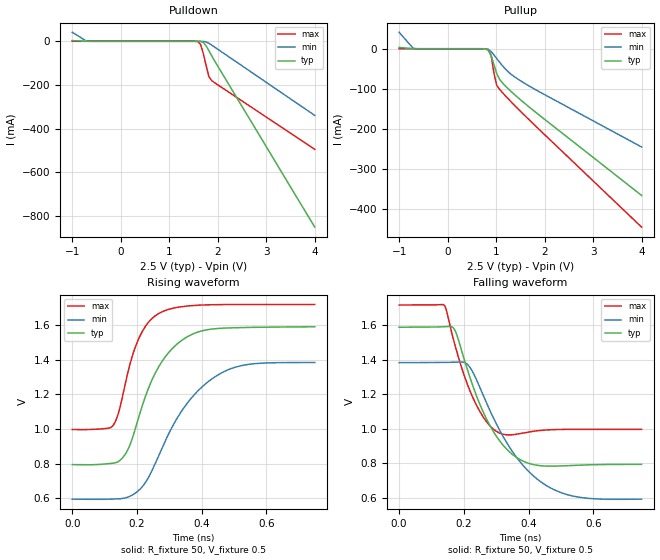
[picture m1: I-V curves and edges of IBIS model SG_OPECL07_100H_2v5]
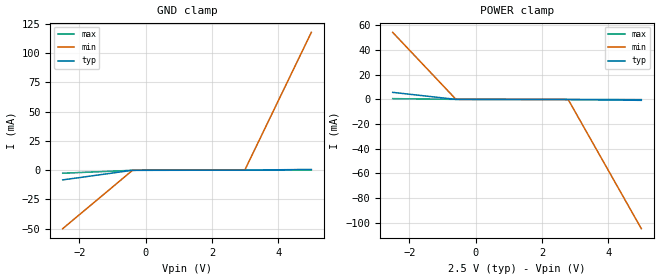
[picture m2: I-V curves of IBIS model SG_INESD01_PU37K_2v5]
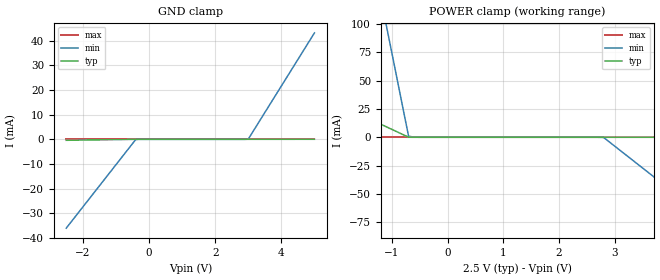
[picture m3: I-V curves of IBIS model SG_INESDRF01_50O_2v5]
|   This file is an IBIS representation of the   |
|   Integrated Device Technology Inc   |
|   8S89874I   |
|   1:2 Differential-to-LVPECL Buffer/Divider   |
[IBIS Ver]   4.1
[File name]   8s89874.ibs
[File Rev]   1.0
[Date]   24 Mar 2011
[Source]   Originated at Integrated Device Technology, Inc.
[Disclaimer]
IDT hereby grants the user of this IBIS model a non-exclusive,
nontransferable license to use this IBIS model under the following terms.
Before using this IBIS model, the user should read this license.
If the user does not accept these terms,  the IBIS model should be
returned to IDT within 30 days.
   The user is granted this license only to use the IBIS model and
is not granted rights to sell, load, rent, lease or license the IBIS
model in whole or in part, or in modified form to anyone other than
user. User may modify the IBIS model to suit its specific
applications but rights to derivative works and such modifications
shall belong to IDT.
   This IBIS model is provided on an "AS IS" basis and IDT makes
absolutely no warranty with respect to the information contained
herein. IDT DISCLAIMS AND CUSTOMER WAIVES ALL WARRANTIES, EXPRESS
OR IMPLIED, INCLUDING WARRANTIES OF MERCHANTABILITY OR FITNESS FOR
A PARTICULAR PURPOSE. The entire risk as to quality and performance
is with the Customer. ACCORDINGLY, IN NO EVENT SHALL THE COMPANY BE
LIABLE FOR ANY DAMAGES, WHETHER IN CONTRACT OR TORT,INCLUDING ANY
LOST PROFITS OR OTHER INCIDENTAL, CONSEQUENTIAL, EXEMPLARY, OR
PUNITIVE DAMAGES ARISING OUT OF THE USE OR APPLICATION OF THE IBIS
model provided in this package. Further, IDT reserves the right to
make changes without notice to any product herein to improve
reliability, function, or design. IDT does not convey any license
under patent rights or any other intellectual property rights,
including those of third parties.
   IDT is not obligated to provide maintenance or support
for the licensed IBIS model.
[Copyright]   Copyright 2011 by IDT Inc.
[Component]   ICS8S89874KI
[Manufacturer] Integrated Device Technology, Inc.
[Package]
|QFN 16
|lead + wire   typ   min   max
R_pkg   72.4655m   58.886m   86.045m
L_pkg   1.47175nH   1.11650nH   1.77850n
C_pkg   0.07747pF   0.07444pF   0.08050pF
[Pin] signal_name  model_name   R_pin   L_pin   C_pin
1   Q0   SG_OPECL07_100H   86.045m   1.77850nH   0.08050pF
2   nQ   SG_OPECL07_100H   58.886m   1.11650nH   0.07444pF
3   Q1   SG_OPECL07_100H   58.886m   1.11650nH   0.07444pF
4   nQ1   SG_OPECL07_100H   86.045m   1.77850nH   0.08050pF
5   S2   SG_INESD01_PU37K   86.045m   1.77850nH   0.08050pF
6   NC   NC   58.886m   1.11650nH   0.07444pF
7   VCC   POWER   58.886m   1.11650nH   0.07444pF
8   nRESET  SG_INESD01_PU37K   86.045m   1.77850nH   0.08050pF
9   nIN   SG_INESDRF01_50O   86.045m   1.77850nH   0.08050pF
10   VREF_AC NC   58.886m   1.11650nH   0.07444pF
11   VT   SG_VTERM02   58.886m   1.11650nH   0.07444pF
12   IN   SG_INESDRF01_50O   86.045m   1.77850nH   0.08050pF
13   VEE   GND   86.045m   1.77850nH   0.08050pF
14   VCC   POWER   58.886m   1.11650nH   0.07444pF
15   S1   SG_INESD01_PU37K   58.886m   1.11650nH   0.07444pF
16   S0   SG_INESD01_PU37K   86.045m   1.77850nH   0.08050pF
[Diff Pin]  inv_pin   vdiff   tdelay_typ   tdelay_min   tdelay_max
|Output
1   2   NA   0   0   0
3   4   NA   0   0   0
|Input
12   9   0.3   0   0   0
[Series Pin Mapping] Pin_2   model_name   function_table_group
12   9   ODT_100
[Model Selector] SG_OPECL07_100H
SG_OPECL07_100H_2v5  Buffer selection for 2v5
SG_OPECL07_100H_3v3  Buffer selection for 3v3
[Model Selector] SG_INESD01_PU37K
SG_INESD01_PU37K_2v5  Buffer selection for 2v5
SG_INESD01_PU37K_3v3  Buffer selection for 3v3
[Model Selector] SG_INESDRF01_50O
SG_INESDRF01_50O_2v5  Buffer selection for 2v5
SG_INESDRF01_50O_3v3  Buffer selection for 3v3
[Model Selector] SG_VTERM02
SG_VTERM02_2v5  Buffer selection for 2v5
SG_VTERM02_3v3  Buffer selection for 3v3
[Model]   ODT_100
Model_type  Series
Polarity   Non-Inverting
|   typ   min   max
C_comp   0pF   0pF   0pF
|   typ   min   max
[Voltage Range]   3.3V   3.135V   3.465V
[R Series]   100ohm   100ohm   100ohm
| Models and submodels in the file (9): ODT_100 (Series), SG_OPECL07_100H_2v5 (Output_ECL), SG_INESD01_PU37K_2v5 (Input), SG_INESDRF01_50O_2v5 (Input), SG_VTERM02_2v5 (Input), SG_OPECL07_100H_3v3 (Output_ECL), SG_INESD01_PU37K_3v3 (Input), SG_INESDRF01_50O_3v3 (Input), SG_VTERM02_3v3 (Input)
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[Model] SG_OPECL07_100H_2v5
Model_type   Output_ECL
Polarity   Non-Inverting
|   typ   min   max
C_comp   2pF   1.5pF   2.5pF
Vmeas = 1.22V
Rref = 50
Cref = 0
Vref = 0.5V
|   typ   min   max
[Voltage range]   2.5V   2.375V   2.625V
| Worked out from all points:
|   rising waveform, R_fixture 50, V_fixture 0.5: 20-80 % time 106ps typ, 147ps min, 70.2ps max; typ from 0.794 V to 1.59 V
|   falling waveform, R_fixture 50, V_fixture 0.5: 20-80 % time 105ps typ, 149ps min, 77.6ps max; typ from 1.59 V to 0.794 V
[Pulldown]
|Voltage   I (typ)   I (min)   I (max)
-999mV    3.236mA    41.07mA    51.47uA
-711.7mV  75.61uA    1.458mA    617.8nA
-654.2mV  8.078uA    226.5uA    35.41nA
1.587V    -86.48uA   -19.21uA   -1.152mA
1.644V    -752.2uA   -118.1uA   -13.49mA
1.702V    -5.318mA   -685.4uA   -55.72mA
1.759V    -20.29mA   -3.152mA   -109.3mA
1.817V    -42.51mA   -9.053mA   -161.7mA
1.874V    -65.92mA   -17.23mA   -179.8mA
4V        -852mA     -339.8mA   -495.5mA
[Pullup]
|Voltage   I (typ)   I (min)   I (max)
-999mV    3.236mA    41.07mA    51.47uA
-711.7mV  75.61uA    1.458mA    617.8nA
724.8mV   -60.94uA   -68.32uA   -5.553uA
839.7mV   -4.039mA   -2.1mA     -1.493mA
897.2mV   -17.48mA   -7.16mA    -16.22mA
954.6mV   -39.41mA   -15.28mA   -60.59mA
1.012V    -62.14mA   -24.41mA   -91.49mA
1.07V     -76.16mA   -33.41mA   -101.1mA
1.127V    -84.99mA   -41.9mA    -109.3mA
1.357V    -112.3mA   -68.3mA    -138.8mA
1.702V    -147.8mA   -94.78mA   -180.2mA
4V        -367.2mA   -246mA     -446.5mA
[Ramp]
|   typ   min   max
dV/dt_r   0.636/0.167n   0.631/0.224n   0.577/0.112n
dV/dt_f   0.649/0.158n   0.638/0.221n   0.605/0.118n
R_load =   50.0000
[Rising Waveform]
R_fixture = 50
V_fixture = 0.5   | VCC_typ - 2V
V_fixture_max = 0.625   | VCC_max - 2V
V_fixture_min = 0.375   | VCC_min - 2V
C_fixture = 0.0p
| Time   typ   min   max
0s        794.1mV    594.5mV    996.6mV
120.9ps   801.1mV    594.9mV    1.011V
154.7ps   831.9mV    598.4mV    1.182V
177.9ps   906.2mV    611.4mV    1.371V
205ps     1.065V     644.6mV    1.519V
271.8ps   1.373V     866.2mV    1.671V
354.4ps   1.531V     1.146V     1.709V
453.5ps   1.58V      1.315V     1.718V
550.3ps   1.586V     1.374V     1.718V
749.2ps   1.589V     1.384V     1.718V
[Falling Waveform]
R_fixture = 50
V_fixture = 0.5   | VCC_typ - 2V
V_fixture_max = 0.625   | VCC_max - 2V
V_fixture_min = 0.375   | VCC_min - 2V
C_fixture = 0.0p
| Time   typ   min   max
0s        1.589V     1.384V     1.718V
138.1ps   1.593V     1.385V     1.719V
167.4ps   1.586V     1.386V     1.521V
219.2ps   1.295V     1.355V     1.218V
263.5ps   1.082V     1.178V     1.058V
306.3ps   940.9mV    1.007V     978.9mV
385.1ps   810.5mV    782.6mV    976.1mV
474.5ps   783.2mV    650.3mV    995.1mV
574.3ps   790.4mV    598.3mV    996.8mV
749.2ps   793.7mV    591.6mV    996.5mV
[Model] SG_INESD01_PU37K_2v5
Model_type   Input
Polarity   Non-Inverting
Vinl = 0.8V
Vinh = 2.2V
|   typ   min   max
C_comp   2pF   1.5pF   2.5pF
|   typ   min   max
[Voltage range]   2.5V   2.375V   2.625V
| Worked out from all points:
|   GND clamp passes 1 mA (typ) near -0.63 V on its own axis
|   POWER clamp passes 1 mA (typ) near -0.92 V on its own axis
[GND_clamp]
|Voltage   I (typ)   I (min)   I (max)
-2.5V     -8.291mA   -49.95mA   -2.608mA
-400mV    -106.4uA   -232.7uA   -107.9uA
3V        15.41uA    485.5uA    13uA
5V        659uA      117.7mA    82.51uA
[Power_clamp]
|Voltage   I (typ)   I (min)   I (max)
-2.5V     5.693mA    54.38mA    628.9uA
-600mV    47.59uA    280.9uA    22.09uA
2.8V      -75.28uA   -402.4uA   -97.1uA
5V        -760.2uA   -104.9mA   -173.7uA
[Model] SG_INESDRF01_50O_2v5
Model_type   Input
Polarity   Non-Inverting
Vinl = 0.8V
Vinh = 2.2V
|   typ   min   max
C_comp   2pF   1.5pF   2.5pF
|   typ   min   max
[Voltage range]   2.5V   2.375V   2.625V
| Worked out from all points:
|   POWER clamp passes 1 mA (typ) near -0.74 V on its own axis
[GND_clamp]
|Voltage   I (typ)   I (min)   I (max)
-2.5V     -396.9uA   -36.05mA   -256.7nA
-400mV    -393.2nA   -69.82uA   -92.43pA
3V        19.97nA    87.82uA    12.78pA
5V        19.18uA    43.19mA    118.6pA
[Power_clamp]
|Voltage   I (typ)   I (min)   I (max)
-2.5V     41.5mA     441.7mA    895.4uA
-1.1V     9.259mA    98.93mA    199.2uA
-1V       6.956mA    74.44mA    149.5uA
-700mV    47.95uA    997.7uA    345.1nA
-500mV    19.97nA    1.53uA     29.89pA
2.8V      -8.026nA   -157uA     -6.301pA
5V        -8.481uA   -84.9mA    -23.18pA
